(* Logix 5000 AddOnInstructionDefinition export VLT_EIP_FC_FLEXIBLE_CTRL; software revision 31.00 *)

TYPE CONTROL_WORD :   // VLT FC Control word
STRUCT
   BIT_00_PRESET_REF_1 : BOOL;   // 0=Reference value, 1=selection lsb
   BIT_01_PRESET_REF_2 : BOOL;   // 0=Reference value, 1=selection msb
   BIT_02_DC_BRAKE_RAMP : BOOL;   // 0=DC brake, 1=Ramp
   BIT_03_COAST_INV : BOOL;   // 0=Coasting, 1=No coasting
   BIT_04_RAMP : BOOL;   // 0=Quick stop, 1=Ramp
   BIT_05_RAMP : BOOL;   // 0=Hold output frequency, 1=Use ramp
   BIT_06_START : BOOL;   // 0=Ramp stop, 1=Start
   BIT_07_RESET : BOOL;   // 0=No function, 1=Reset
   BIT_08_JOG : BOOL;   // 0=No function, 1=Jog
   BIT_09_RAMP_1_2 : BOOL;   // 0=Ramp 1, 1=Ramp 2
   BIT_10_USE_CTRL_WORD : BOOL;   // 0=Dont use CTW, 1= Use CTW
   BIT_11_RLY_1_ON : BOOL;   // 0=Relay 01 deactived, 1=Relay 01 active
   BIT_12_RLY_2_ON : BOOL;   // 0=Relay 02 deactived, 1=Relay 02 active
   BIT_13_SETUP_SEL_1 : BOOL;   // 0=Parameter set-up, 1=selection lsb
   BIT_14_SETUP_SEL_2 : BOOL;   // 0=Parameter set-up, 1=selection msb
   BIT_15_REVERSE : BOOL;   // 0= No Reverse, 1= Reverse
END_STRUCT
END_TYPE

TYPE FLEXI_CTRL_VLT_IN_DDT :   // Input data read structure. Holds the data structure obtained from the Process data (PCDREAD) and expressed in user data accessible format
STRUCT
   STW : STATUS_WORD;   // Status word
   MAV : INT;   // Main actual value (Speed) in raw. -16384 to +16384
   PCD_02 : INT;   // Depends on Drive config.
   PCD_03 : INT;   // Depends on Drive config.
   PCD_04 : INT;   // Depends on Drive config.
   PCD_05 : INT;   // Depends on Drive config.
   PCD_06 : INT;   // Depends on Drive config.
   PCD_07 : INT;   // Depends on Drive config.
   PCD_08 : INT;   // Depends on Drive config.
   PCD_09 : INT;   // Depends on Drive config.
END_STRUCT
END_TYPE

TYPE FLEXI_CTRL_VLT_OUT_DDT :   // Output write data structure. Holds the data structure in user data accessible format to send the Process data (PCDWRITE) to the frerquency converter.
STRUCT
   CTW : CONTROL_WORD;   // Control word
   MRV : INT;   // Main reference value (Speed) in raw. -16384 to +16384
   PCD_02 : INT;   // Depends on Drive config
   PCD_03 : INT;   // Depends on Drive config
   PCD_04 : INT;   // Depends on Drive config
   PCD_05 : INT;   // Depends on Drive config
   PCD_06 : INT;   // Depends on Drive config
   PCD_07 : INT;   // Depends on Drive config
   PCD_08 : INT;   // Depends on Drive config
   PCD_09 : INT;   // Depends on Drive config
END_STRUCT
END_TYPE

TYPE STATUS_WORD :   // VLT FC Status word
STRUCT
   BIT_00_CTRL_RDY : BOOL;   // 0=Control not ready, 1=Control ready
   BIT_01_DRV_RDY : BOOL;   // 0=Frequency converter, 1=Frequency converter ready
   BIT_02_COAST_RDY : BOOL;   // 0=Coasting, 1=Enable
   BIT_03_TRIP : BOOL;   // 0=No error, 1=Trip
   BIT_04_ERROR : BOOL;   // 0=No error, 1=Error (no trip)
   BIT_05_RESERVED : BOOL;   // 0=Reserved, 1=---
   BIT_06_TRIPLOCK : BOOL;   // 0=No error, 1=Triplock
   BIT_07_WARNING : BOOL;   // 0=No warning, 1=Warning
   BIT_08_RUNNING_REF : BOOL;   // 0=Speed <> reference, 1=Speed=reference
   BIT_09_CTRL_SOURCE : BOOL;   // 0=Local operation, 1=Bus control
   BIT_10_F_LIMIT_OK : BOOL;   // 0=Out of frequency limit, 1=Frequency limit ok
   BIT_11_IN_OPR : BOOL;   // 0=No operation, 1=In operation
   BIT_12_IN_AUTOSTART : BOOL;   // 0=Frequency converter OK, 1=Stopped, autostart
   BIT_13_VOLT_MAX : BOOL;   // 0=Voltage OK, 1=Voltage exceeded
   BIT_14_TORQ_MAX : BOOL;   // 0=Torque OK, 1=Torque exceeded
   BIT_15_TIMER_EXD : BOOL;   // 0=Timer OK, 1=Timer exceeded
END_STRUCT
END_TYPE

ADD_ON_INSTRUCTION VLT_EIP_FC_FLEXIBLE_CTRL   (* revision 1.0, vendor Danfoss Drives *)
// Flexible Control Add-On instruction for Danfoss FC series Drives
VAR_INPUT
   FB_CTRL_EN : BOOL; {visible}   // Bit 10. 0 = Data Invalid, 1 = Data Valid
   PRESET_REF_1 : BOOL; {visible}   // Bit 0. 0 = Reference value, 1 = Selection LSB
   PRESET_REF_2 : BOOL; {visible}   // Bit 1. 0 = Reference value, 1 = Selection MSB
   DC_BRAKE_RAMP : BOOL := 1; {visible}   // Bit 2. 0 = DC brake, 1 = Ramp
   COAST_INV : BOOL := 1; {visible}   // Bit 3. 0 = Coasting, 1 = No coasting
   QSTP_RMP : BOOL := 1; {visible}   // Bit 4. 0 = Quick stop, 1 = Ramp
   HLD_RMP : BOOL := 1; {visible}   // Bit 5. 0 = Hold output frequency, 1 = Use ramp
   START : BOOL; {visible}   // Bit 6. 0 = Ramp stop, 1 = Start
   RESET : BOOL; {visible}   // Bit 7. 0 = No function, 1 = Reset
   JOG : BOOL; {visible}   // Bit 8. 0 = No function, 1 = Jog
   RAMP_1_2 : BOOL; {visible}   // Bit 9. 0 = Ramp 1, 1 = Ramp 2
   RLY_1_ON : BOOL; {visible}   // Bit 11. 0 = Relay 01 deactivated, 1 = Relay 01 active
   RLY_2_ON : BOOL; {visible}   // Bit 12. 0 = Relay 02 deactivated, 1 = Relay 02 active
   SETUP_SEL_1 : BOOL; {visible}   // Bit 13. 0 = Parameter set-up, 1 = Selection LSB
   SETUP_SEL_2 : BOOL; {visible}   // Bit 14. 0 = Parameter set-up, 1 = Selection MSB
   REVERSE : BOOL; {visible}   // Bit 15. 0 = No reverse, 1 = Reverse
   REF_VALUE : INT; {visible}   // Drive Ref. -16384 to +16384
   COMM_STATUS : BOOL; {required}   // Communication status
END_VAR
VAR_OUTPUT
   READY : BOOL; {access Read Only, visible}   // Ready for operation
   FAULT : BOOL; {access Read Only, visible}   // Alarm pending
   WARNING : BOOL; {access Read Only, visible}   // Warning pending
   RUNNING : BOOL; {access Read Only, visible}   // Motor engaged
   RUN_ON_REF : BOOL; {access Read Only, visible}   // Speed = reference
   COMM_OK : BOOL; {access Read Only, visible}   // Communication OK
   MAV : INT; {access Read Only, visible}   // Main actual value
END_VAR
VAR_IN_OUT
   PCDREAD : INT[10]; {required}   // Process data from Drive
        [0]   // Status word
        [1]   // Main actual value
        [2]   // Depends on Drive config.
        [3]   // Depends on Drive config.
        [4]   // Depends on Drive config.
        [5]   // Depends on Drive config.
        [6]   // Depends on Drive config.
        [7]   // Depends on Drive config.
        [8]   // Depends on Drive config.
        [9]   // Depends on Drive config.
   PCDWRITE : INT[10]; {required}   // Process data to Drive
        [0]   // Control word
        [1]   // Main reference value
        [2]   // Depends on Drive config.
        [3]   // Depends on Drive config.
        [4]   // Depends on Drive config.
        [5]   // Depends on Drive config.
        [6]   // Depends on Drive config.
        [7]   // Depends on Drive config.
        [8]   // Depends on Drive config.
        [9]   // Depends on Drive config.
   DATA_READ : FLEXI_CTRL_VLT_IN_DDT; {required}   // Process read data in User defined structure
        .STW   // Status word
        .MAV   // Main actual value
        .PCD_02   // Depends on Drive config.
        .PCD_03   // Depends on Drive config.
        .PCD_04   // Depends on Drive config.
        .PCD_05   // Depends on Drive config.
        .PCD_06   // Depends on Drive config.
        .PCD_07   // Depends on Drive config.
        .PCD_08   // Depends on Drive config.
        .PCD_09   // Depends on Drive config.
   DATA_WRITE : FLEXI_CTRL_VLT_OUT_DDT; {required}   // Process write data in User defined structure
        .CTW   // Control word
        .MRV   // Main reference value
        .PCD_02   // Depends on Drive config.
        .PCD_03   // Depends on Drive config.
        .PCD_04   // Depends on Drive config.
        .PCD_05   // Depends on Drive config.
        .PCD_06   // Depends on Drive config.
        .PCD_07   // Depends on Drive config.
        .PCD_08   // Depends on Drive config.
        .PCD_09   // Depends on Drive config.
END_VAR
VAR
   AUX_VALUE : DINT; {access None}   // Internal variable - Main Actual Value( Raw value)
END_VAR

ROUTINE Logic   (* structured text *)
   //Communication health status
   COMM_OK := NOT COMM_STATUS;
   
   // Read Operation
   // Copying Status word from PCDREAD [0] to user accessible data structure
   DATA_READ.STW.BIT_00_CTRL_RDY := PCDREAD[0].0;
   DATA_READ.STW.BIT_01_DRV_RDY := PCDREAD[0].1;
   DATA_READ.STW.BIT_02_COAST_RDY := PCDREAD[0].2;
   DATA_READ.STW.BIT_03_TRIP := PCDREAD[0].3;
   DATA_READ.STW.BIT_04_ERROR := PCDREAD[0].4;
   DATA_READ.STW.BIT_05_RESERVED := PCDREAD[0].5;
   DATA_READ.STW.BIT_06_TRIPLOCK := PCDREAD[0].6;
   DATA_READ.STW.BIT_07_WARNING := PCDREAD[0].7;
   DATA_READ.STW.BIT_08_RUNNING_REF := PCDREAD[0].8;
   DATA_READ.STW.BIT_09_CTRL_SOURCE := PCDREAD[0].9;
   DATA_READ.STW.BIT_10_F_LIMIT_OK := PCDREAD[0].10;
   DATA_READ.STW.BIT_11_IN_OPR := PCDREAD[0].11;
   DATA_READ.STW.BIT_12_IN_AUTOSTART := PCDREAD[0].12;
   DATA_READ.STW.BIT_13_VOLT_MAX := PCDREAD[0].13;
   DATA_READ.STW.BIT_14_TORQ_MAX := PCDREAD[0].14;
   DATA_READ.STW.BIT_15_TIMER_EXD := PCDREAD[0].15;
   
   // Copying MAV data, PCDREAD [2]..PCDREAD [9] to user accessible data structure
   DATA_READ.MAV := PCDREAD[1];
   DATA_READ.PCD_02 := PCDREAD[2];
   DATA_READ.PCD_03 := PCDREAD[3];
   DATA_READ.PCD_04 := PCDREAD[4];
   DATA_READ.PCD_05 := PCDREAD[5];
   DATA_READ.PCD_06 := PCDREAD[6];
   DATA_READ.PCD_07 := PCDREAD[7];
   DATA_READ.PCD_08 := PCDREAD[8];
   DATA_READ.PCD_09 := PCDREAD[9];
   
   // Write Operation
   // Copying MRV and user accessible data structure to Process data write channel
   DATA_WRITE.MRV := REF_VALUE;
   
   // Mapping inputs to InOut parameter
   DATA_WRITE.CTW.BIT_00_PRESET_REF_1 := PRESET_REF_1;
   DATA_WRITE.CTW.BIT_01_PRESET_REF_2 := PRESET_REF_2;
   DATA_WRITE.CTW.BIT_02_DC_BRAKE_RAMP := DC_BRAKE_RAMP;
   DATA_WRITE.CTW.BIT_03_COAST_INV := COAST_INV;
   DATA_WRITE.CTW.BIT_04_RAMP := QSTP_RMP;
   DATA_WRITE.CTW.BIT_05_RAMP := HLD_RMP;
   DATA_WRITE.CTW.BIT_06_START := START;
   DATA_WRITE.CTW.BIT_07_RESET := RESET;
   DATA_WRITE.CTW.BIT_08_JOG := JOG;
   DATA_WRITE.CTW.BIT_09_RAMP_1_2 := RAMP_1_2;
   DATA_WRITE.CTW.BIT_10_USE_CTRL_WORD := FB_CTRL_EN;		//If BIT_10_USE_CTRL_WORD is FALSE then there is no Drive control from teh fieldbus possible
   DATA_WRITE.CTW.BIT_11_RLY_1_ON := RLY_1_ON;
   DATA_WRITE.CTW.BIT_12_RLY_2_ON := RLY_2_ON;
   DATA_WRITE.CTW.BIT_13_SETUP_SEL_1 := SETUP_SEL_1;
   DATA_WRITE.CTW.BIT_14_SETUP_SEL_2 := SETUP_SEL_2;
   DATA_WRITE.CTW.BIT_15_REVERSE := REVERSE;
   
   // Copying Control word from PCDWRITE [0] to user accessible data structure
   PCDWRITE[0].0 := DATA_WRITE.CTW.BIT_00_PRESET_REF_1;
   PCDWRITE[0].1 := DATA_WRITE.CTW.BIT_01_PRESET_REF_2;
   PCDWRITE[0].2 := DATA_WRITE.CTW.BIT_02_DC_BRAKE_RAMP;
   PCDWRITE[0].3 := DATA_WRITE.CTW.BIT_03_COAST_INV;
   PCDWRITE[0].4 := DATA_WRITE.CTW.BIT_04_RAMP;
   PCDWRITE[0].5 := DATA_WRITE.CTW.BIT_05_RAMP;
   PCDWRITE[0].6 := DATA_WRITE.CTW.BIT_06_START;
   PCDWRITE[0].7 := DATA_WRITE.CTW.BIT_07_RESET;
   PCDWRITE[0].8 := DATA_WRITE.CTW.BIT_08_JOG;
   PCDWRITE[0].9 := DATA_WRITE.CTW.BIT_09_RAMP_1_2;
   PCDWRITE[0].10 := DATA_WRITE.CTW.BIT_10_USE_CTRL_WORD;
   PCDWRITE[0].11 := DATA_WRITE.CTW.BIT_11_RLY_1_ON;
   PCDWRITE[0].12 := DATA_WRITE.CTW.BIT_12_RLY_2_ON;
   PCDWRITE[0].13 := DATA_WRITE.CTW.BIT_13_SETUP_SEL_1;
   PCDWRITE[0].14 := DATA_WRITE.CTW.BIT_14_SETUP_SEL_2;
   PCDWRITE[0].15 := DATA_WRITE.CTW.BIT_15_REVERSE;
   
   // Copying MRV and user accessible data structure to Process data write channel
   PCDWRITE[1] := DATA_WRITE.MRV;
   PCDWRITE[2] := DATA_WRITE.PCD_02;
   PCDWRITE[3] := DATA_WRITE.PCD_03;
   PCDWRITE[4] := DATA_WRITE.PCD_04;
   PCDWRITE[5] := DATA_WRITE.PCD_05;
   PCDWRITE[6] := DATA_WRITE.PCD_06;
   PCDWRITE[7] := DATA_WRITE.PCD_07;
   PCDWRITE[8] := DATA_WRITE.PCD_08;
   PCDWRITE[9] := DATA_WRITE.PCD_09;
   
   //Communication health statusbV
   READY := (DATA_READ.STW.BIT_00_CTRL_RDY & 											(* 1 = Control Ready *)
   		  DATA_READ.STW.BIT_01_DRV_RDY & 											(* 1 = Frequency converter ready *)
   		  DATA_READ.STW.BIT_02_COAST_RDY & 											(* 1 = Costing stop *)
   		  DATA_READ.STW.BIT_09_CTRL_SOURCE &										(* 1 = Bus control *)
   		  COMM_OK);																	(* 1 = Communication between device and PLC is healthy *)
   FAULT := (DATA_READ.STW.BIT_03_TRIP OR 												(* 1 = The frequency converter trips *)
   		  DATA_READ.STW.BIT_04_ERROR OR  											(* 1 = The frequency converter shows an error but does not trip. *)
   		  DATA_READ.STW.BIT_06_TRIPLOCK OR	  										(* 1 = The frequency converter is tripped and locked *)
   		  NOT COMM_OK);																(* 1 = Communication failure *)
   WARNING := DATA_READ.STW.BIT_07_WARNING & COMM_OK;  								(* 1 = A warning has occurred on the drive *)
   RUNNING := DATA_READ.STW.BIT_11_IN_OPR & COMM_OK; 									(* 1 = The frequency converter has a start signal or the output frequency is and greater than 0 Hz.*)
   RUN_ON_REF := DATA_READ.STW.BIT_08_RUNNING_REF AND COMM_OK;							(* 1 = The actual motor speed reaches the preset speed reference *)
   MAV := DATA_READ.MAV;
END_ROUTINE
END_ADD_ON_INSTRUCTION
